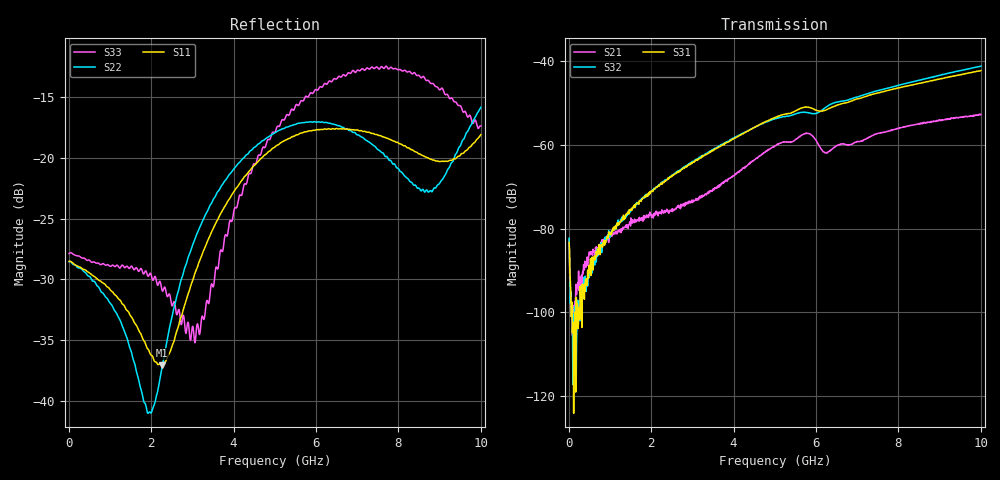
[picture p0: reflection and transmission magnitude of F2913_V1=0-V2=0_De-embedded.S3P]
! Integrated Device Technology
! Corporate Headquarters
! 6024 Silver Creek Valley Road
! San Jose, CA 95138  USA
! Phone:  1-408-284-8200
! Toll Free:  1-800-223-1366
! Webpage:  http://www.idt.com/
! Timing and RF Division
! 515 Groton Road, Suite 102
! Westford, MA 01886-6024
! Device:  F2913
! Description: High Isolation SP2T RF Switch
! Frequency:  0.050 -  6.000 GHz
! Package:  4x4 mm QFN Plastic Package: 20 pin
! Ports:  3 RF, 3 DC
!  Pin  1  = GND
!  Pin  2  = GND
!  Pin  3  = RF1  =  Port 1
!  Pin  4  = GND
!  Pin  5  = GND
!  Pin  6  = GND
!  Pin  7  = GND
!  Pin  8  = RFC  =  Port 3
!  Pin  9  = GND
!  Pin 10  = GND
!  Pin 11  = GND
!  Pin 12  = GND
!  Pin 13  = RF2  =  Port 2
!  Pin 14  = GND
!  Pin 15  = GND
!  Pin 16  = C2
!  Pin 17  = C1
!  Pin 18  = GND
!  Pin 19  = GND
!  Pin 20  = Vdd
! State:  Both Paths not selected
! C1:  0.0 V (Logic Low)
! C2:  0.0 V (Logic Low)
! Voltage:  +3.30  Volts
! Current:  0.082 mA
! Data:  The device was measured on a F2913 evaluation board which has
!  individual transmission lines to the RF pins.  Data was collected
!  using a calibrated network analyzer.  The evaluation board was
!  de-embedded using a AFR (Keysight Technologies).
!  The reference plane is the edge of the package pin.
! Misc:
!  Action Tracker AT0430
!  WorkFront Reference Number 1053824
! Date Measured:  2018-08-23
! Date:  2018-08-24  MJV
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# Hz S dB R 50
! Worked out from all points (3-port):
!   1000 points, 10 MHz to 10 GHz, reference 50 ohm
!   strongest paths, dB at 10 MHz, 2.51 GHz, 5.01 GHz, 7.51 GHz, 10 GHz:
!     S31: -83.3, -67.5, -53.4, -47.6, -42.3
!     S32: -82.3, -67.3, -53.7, -47.0, -41.2
!     S21: -82.5, -75.3, -60.2, -57.2, -52.8
!   lowest |S11| = -37.1 dB at 2.26 GHz (marker M1), VSWR 1.03, Z = 49.1 + j1.08 ohm
!   |S11| at or under -10 dB: start of sweep to end of sweep
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1e7  -28.51 -179.8  -83.12 -39.7  -82.78 -47.5
     -82.52 -43.9  -28.54 -179.7  -82.56 -39.9
     -83.30 -45.8  -82.30 -47.5  -27.89 -179.3
1.11e9  -31.23 173.4  -81.34 79.6  -80.11 134.9
        -80.92 75.8  -32.52 176.0  -80.20 125.6
        -79.62 127.9  -80.27 130.3  -28.93 -152.9
1.94e9  -35.78 155.4  -77.23 84.7  -71.42 135.6
        -77.31 83.9  -40.93 127.3  -71.65 137.8
        -71.42 137.7  -71.49 137.8  -29.72 -135.9
2.26e9  -37.06 128.6  -76.30 85.7  -69.14 135.0
        -75.50 84.2  -37.33 80.0  -69.36 136.9
        -69.23 137.1  -68.87 138.1  -30.83 -131.3
3.09e9  -29.26 85.4  -72.84 101.5  -63.62 137.3
        -72.80 97.7  -26.42 69.7  -63.46 137.0
        -63.59 137.5  -63.56 137.4  -34.42 179.8
5.01e9  -19.10 105.8  -60.10 93.3  -53.42 116.6
        -60.15 93.2  -17.94 103.1  -53.75 114.4
        -53.41 116.9  -53.71 114.5  -17.89 143.6
5.8e9  -17.84 116.0  -57.26 58.9  -51.01 96.8
       -57.27 59.4  -17.09 116.2  -52.30 101.0
       -51.00 96.8  -52.30 100.8  -15.03 151.7
6.26e9  -17.68 120.4  -61.86 55.8  -51.60 97.8
        -61.81 55.4  -17.12 122.6  -50.87 107.0
        -51.57 97.7  -50.87 107.1  -13.99 155.7
8.77e9  -20.11 106.5  -54.48 42.8  -44.78 71.9
        -54.54 42.4  -22.72 84.8  -43.89 74.0
        -44.72 72.0  -43.95 73.6  -13.87 167.8
1e10  -18.12 62.2  -52.75 22.8  -42.27 54.5
      -52.80 24.0  -15.86 39.6  -41.20 53.2
      -42.27 54.2  -41.19 53.1  -17.39 139.6
